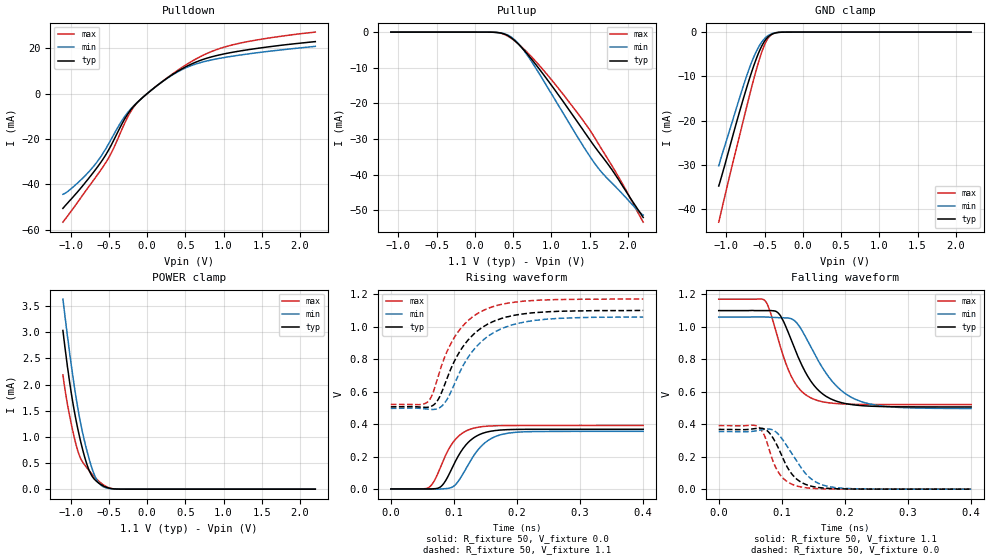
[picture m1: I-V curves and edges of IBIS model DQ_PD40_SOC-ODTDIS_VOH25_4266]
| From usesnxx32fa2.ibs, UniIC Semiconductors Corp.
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| DQ_PD40_SOC-ODTDIS_VOH25_4266
| (40 Ohm Pulldown, SOC ODT disabled setting, VOH=VDDQ/2.5 cal. point, 3200-4266Mbps)
[Model]   DQ_PD40_SOC-ODTDIS_VOH25_4266
Model_type   I/O
Vinl = 160.000mV
Vinh = 280.000mV
Vmeas = 220.000mV
Vref = 0.0mV
Cref = 0.0pF
|   typ   min   max
|C_comp   0.834pF   0.784pF   0.884pF
C_comp_pullup   0.4170pF   0.3920pF   0.4420pF
C_comp_pulldown   0.4170pF   0.3920pF   0.4420pF
| Note: C_comp changes when the ODT circuit is enabled.
[Model Spec]
| Input threshold voltage corners
Vinl   0.1600V   0.1520V   0.1740V
Vinh   0.2800V   0.2720V   0.2940V
| Measurement voltage corners
Vmeas   0.2200V   0.2120V   0.2340V
| Timing spec test load voltage corners
Vref   0.0000V   0.0000V   0.0000V
| Dynamic Overshoot Parameters from LPDDR4 Specification
D_overshoot_ampl_h   0.30   NA   NA
D_overshoot_ampl_l   0.30   NA   NA
D_overshoot_area_h   0.1n   NA   NA
D_overshoot_area_l   0.1n   NA   NA
[Voltage Range]   1.1000V   1.0600V   1.1700V
[Pullup Reference]   1.1000V   1.0600V   1.1700V
| Junction Temperature (Ambient temp is 35C typ 95C min -40C max)
[Temperature Range]   50.0   110.0   -40.0
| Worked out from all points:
|   slope of the pulldown table from 0 to 0.165 V, typ, clamps not added: 36.9 ohm
|   slope of the pullup table from 0 to 0.165 V, typ, clamps not added: 17.1 kohm
|   GND clamp passes 1 mA (typ) near -0.45 V on its own axis
|   POWER clamp passes 1 mA (typ) near -0.88 V on its own axis
|   rising waveform, R_fixture 50, V_fixture 0.0: 20-80 % time 34.6ps typ, 38.2ps min, 31.6ps max; typ from 0.001 V to 0.368 V
|   falling waveform, R_fixture 50, V_fixture 1.1: 20-80 % time 45.6ps typ, 57.6ps min, 35.8ps max; typ from 1.1 V to 0.507 V
|   rising waveform, R_fixture 50, V_fixture 1.1: 20-80 % time 56.3ps typ, 59.8ps min, 51.7ps max; typ from 0.507 V to 1.1 V
|   falling waveform, R_fixture 50, V_fixture 0.0: 20-80 % time 31.3ps typ, 39.3ps min, 25.3ps max; typ from 0.368 V to 0.001 V
[Pulldown]
|   Voltage   I(typ)   I(min)   I(max)
-1.1V     -50.64mA   -44.42mA   -56.73mA
-915.2mV  -43.62mA   -39.66mA   -48.31mA
-684.2mV  -33.99mA   -31.46mA   -37.48mA
-482.9mV  -23.65mA   -20.99mA   -27.19mA
-317.9mV  -12.72mA   -11.35mA   -14.94mA
-179.3mV  -5.752mA   -5.546mA   -6.132mA
-60.5mV   -1.802mA   -1.786mA   -1.779mA
229.9mV   6.063mA    5.989mA    6.147mA
569.8mV   12.91mA    12.29mA    13.97mA
952.6mV   17.16mA    15.62mA    19.95mA
1.418V    19.88mA    17.97mA    23.61mA
2.2V      22.98mA    20.89mA    27.18mA
[GND Clamp]
|   Voltage   I(typ)   I(min)   I(max)
-1.1V     -34.75mA   -30.2mA    -42.92mA
-1.027V   -30.44mA   -26.03mA   -37.57mA
-941.6mV  -25.02mA   -21.25mA   -31.33mA
-793.1mV  -15.92mA   -12.96mA   -20.97mA
-667.7mV  -8.911mA   -6.72mA    -12.3mA
-595.1mV  -5.401mA   -3.898mA   -7.695mA
-525.8mV  -2.771mA   -1.974mA   -3.966mA
-469.7mV  -1.358mA   -985.2uA   -1.787mA
-416.9mV  -597.2uA   -440.2uA   -665.5uA
-354.2mV  -179uA     -134.5uA   -160.5uA
-258.5mV  -16.23uA   -14.39uA   -9.948uA
2.2V      0A         0A         0A
[Pullup]
|   Voltage   I(typ)   I(min)   I(max)
-1.1V     4.106uA    7.431uA    1.361uA
256.3mV   -57.83uA   -56.08uA   -56.76uA
394.9mV   -631.3uA   -523.9uA   -750.6uA
503.8mV   -2.099mA   -1.888mA   -2.196mA
606.1mV   -4.22mA    -4.209mA   -4.061mA
741.4mV   -7.628mA   -8.301mA   -6.975mA
1.065V    -16.85mA   -19.63mA   -15.08mA
1.461V    -28.96mA   -33.53mA   -26.23mA
1.609V    -33.42mA   -38.12mA   -31.2mA
1.698V    -35.91mA   -40.36mA   -34.29mA
1.887V    -41.73mA   -44.49mA   -41mA
2.2V      -52.05mA   -51.39mA   -53.39mA
[POWER Clamp]
|   Voltage   I(typ)   I(min)   I(max)
-1.1V     3.033mA    3.633mA    2.184mA
-1.041V   2.345mA    2.929mA    1.625mA
-981.2mV  1.753mA    2.275mA    1.183mA
-911.9mV  1.2mA      1.61mA     764.6uA
-852.5mV  818.1uA    1.148mA    543.5uA
-776.6mV  434.1uA    683.2uA    390.2uA
-707.3mV  225.4uA    345.4uA    267.6uA
-651.2mV  138.6uA    162.4uA    181.2uA
-591.8mV  77.93uA    64.79uA    105.5uA
-489.5mV  17.84uA    10.81uA    22.44uA
-367.4mV  1.189uA    872.9nA    943.4nA
2.2V      0A         0A         0A
[Ramp]
|   typ   min   max
| 20% - 80%
dV/dt_r   220.67m/34.62p   212.99m/38.16p   234.73m/31.58p
dV/dt_f   356.03m/45.65p   337.71m/57.58p   389.19m/35.75p
| 25% - 75%
|dV/dt_r   183.89m/27.56p   177.50m/30.42p   195.60m/25.07p
|dV/dt_f   296.69m/36.41p   281.42m/45.98p   324.32m/28.47p
R_load = 50
[Rising Waveform]
R_fixture = 50
V_fixture = 0.0
|   Time   V(typ)   V(min)   V(max)
0s        576.2uV    460uV      427uV
59ps      302.1uV    60.2uV     6.861mV
68ps      1.699mV    -527.5uV   44.07mV
78ps      11.14mV    298.1uV    126.8mV
103ps     173.9mV    28.19mV    307.8mV
117ps     261.2mV    109.9mV    352.6mV
132ps     316.6mV    207.5mV    375.5mV
156ps     354.2mV    303.3mV    388.2mV
188ps     366.4mV    345.1mV    391.3mV
401ps     368.4mV    355.4mV    391.6mV
[Falling Waveform]
R_fixture   = 50
V_fixture   = 1.1
V_fixture_min = 1.06
V_fixture_max = 1.17
|   Time   V(typ)   V(min)   V(max)
0s        1.1V       1.06V      1.17V
74ps      1.1V       1.06V      1.159V
96ps      1.079V     1.056V     903.5mV
115ps     920.8mV    1.05V      697.3mV
128ps     797.9mV    1.004V     618.1mV
149ps     651.2mV    856.1mV    557.7mV
184ps     546.5mV    648mV      528.4mV
223ps     516mV      544.4mV    522.5mV
279ps     507.9mV    505.4mV    521.5mV
401ps     506.6mV    497.1mV    521.4mV
[Rising Waveform]
R_fixture   = 50
V_fixture   = 1.1
V_fixture_min = 1.06
V_fixture_max = 1.17
|   Time   V(typ)   V(min)   V(max)
0s        506.5mV    496.8mV    521.3mV
57ps      503.2mV    492.6mV    532.3mV
66ps      513.1mV    490.1mV    582.9mV
79ps      579.9mV    504.6mV    741.8mV
94ps      727.7mV    586.1mV    885.4mV
112ps     862.2mV    739.3mV    993.7mV
130ps     947.6mV    849.8mV    1.06V
152ps     1.011V     933.9mV    1.109V
227ps     1.086V     1.038V     1.161V
401ps     1.1V       1.059V     1.17V
[Falling Waveform]
R_fixture = 50
V_fixture = 0.0
|   Time   V(typ)   V(min)   V(max)
0s        368.5mV    355.6mV    391.7mV
58ps      374mV      358.9mV    392.3mV
75ps      365.9mV    370.3mV    307.4mV
86ps      317mV      364.6mV    174.7mV
96ps      243.4mV    333.4mV    97.47mV
111ps     122.2mV    250.2mV    41.27mV
126ps     55.84mV    161.1mV    17.92mV
150ps     16.22mV    54.74mV    5.098mV
181ps     3.876mV    12.57mV    1.335mV
401ps     621.2uV    531.5uV    445.4uV
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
